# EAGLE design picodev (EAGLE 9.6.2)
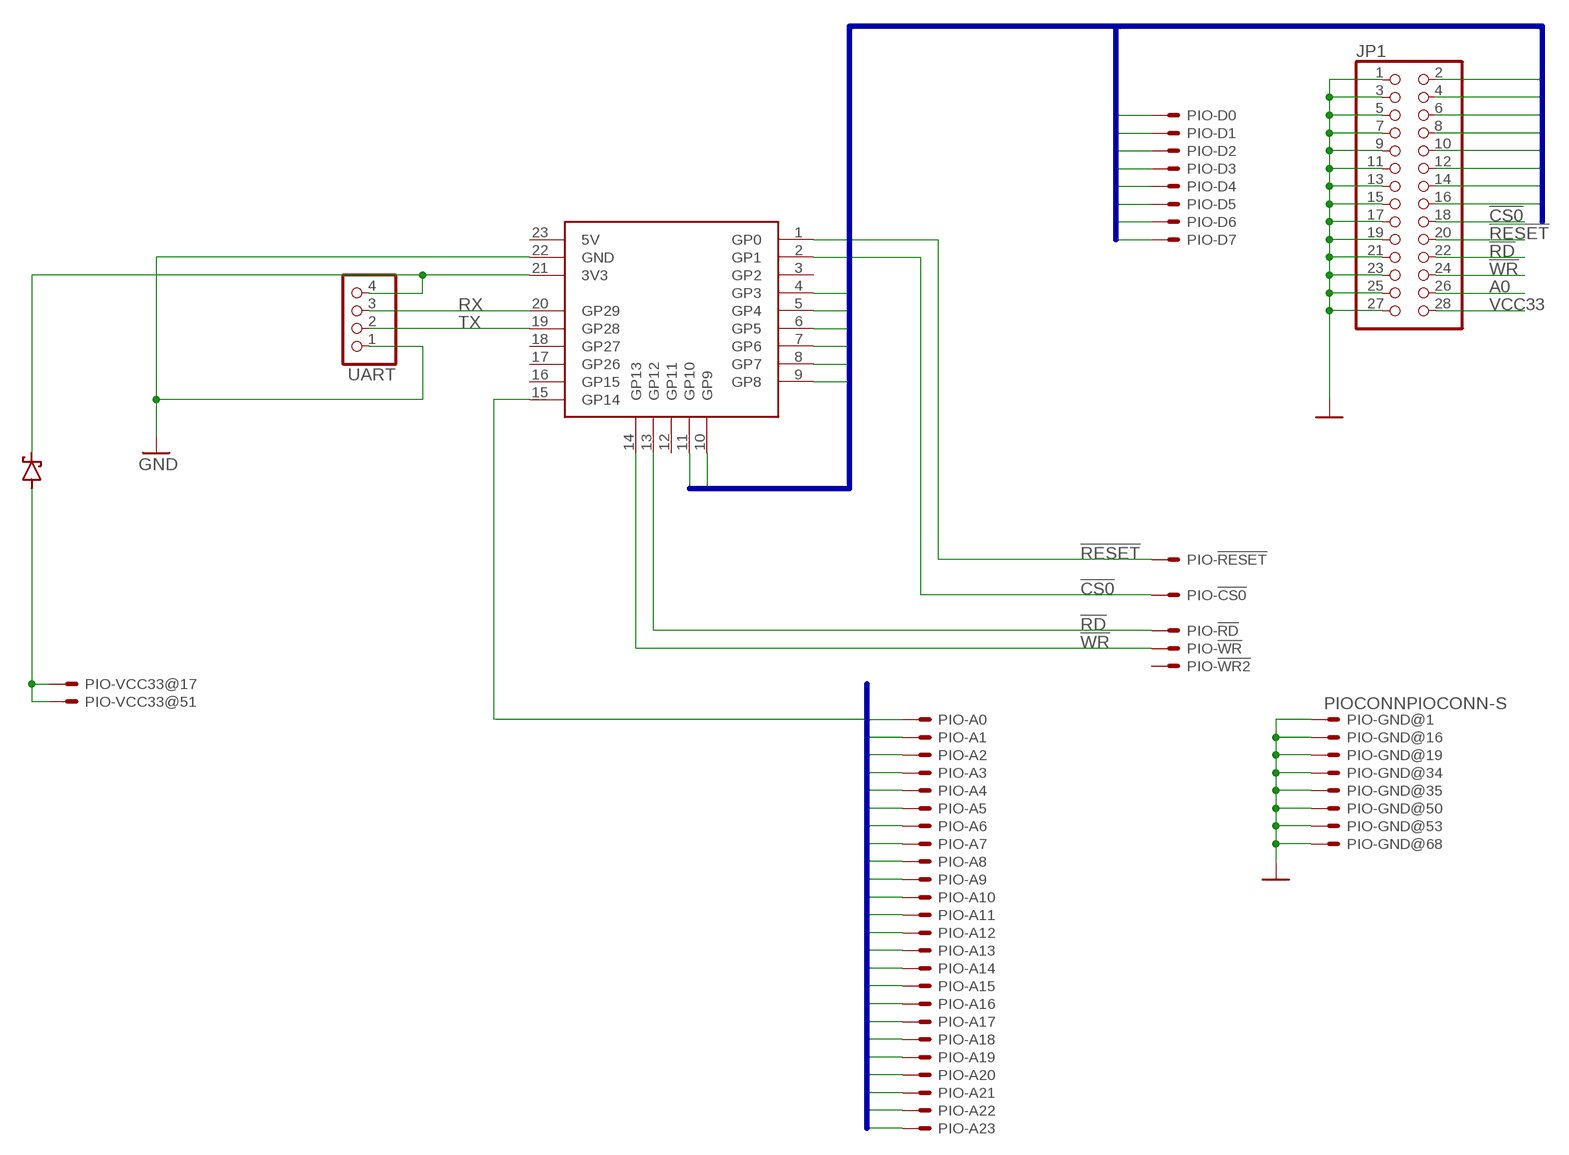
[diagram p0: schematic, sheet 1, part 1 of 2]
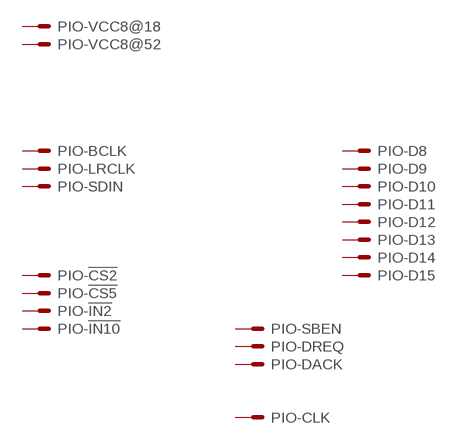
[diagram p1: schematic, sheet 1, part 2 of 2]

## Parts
D  SCHOTTKYSMA  [SMADIODE]
JP1  PINHD-2X14  [2X14]
PIO  PIOCONNPIOCONN-S  [PIOCONN]
U$1  PICO-ZERO  [PICO-ZERO]
UART  PINHD-1X4  [1X04]

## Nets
!CS0: JP1.18 PIO.4 U$1.2(GP1)
!RD: JP1.22 PIO.30 U$1.13(GP12)
!RESET: JP1.20 PIO.2 U$1.1(GP0)
!WR: JP1.24 PIO.64 U$1.14(GP13)
A0: JP1.26 PIO.14 U$1.15(GP14)
A1: PIO.48
A2: PIO.15
A3: PIO.49
A4: PIO.20
A5: PIO.54
A6: PIO.21
A7: PIO.55
A8: PIO.22
A9: PIO.56
A10: PIO.23
A11: PIO.57
A12: PIO.24
A13: PIO.58
A14: PIO.25
A15: PIO.59
A16: PIO.26
A17: PIO.60
A18: PIO.27
A19: PIO.61
A20: PIO.28
A21: PIO.62
A22: PIO.29
A23: PIO.63
D0: JP1.16 PIO.6 U$1.4(GP3)
D1: JP1.14 PIO.40 U$1.5(GP4)
D2: JP1.12 PIO.7 U$1.6(GP5)
D3: JP1.10 PIO.41 U$1.7(GP6)
D4: JP1.8 PIO.8 U$1.8(GP7)
D5: JP1.6 PIO.42 U$1.9(GP8)
D6: JP1.4 PIO.9 U$1.10(GP9)
D7: JP1.2 PIO.43 U$1.11(GP10)
GND: JP1.1 JP1.3 JP1.5 JP1.7 JP1.9 JP1.11 JP1.13 JP1.15 JP1.17 JP1.19 JP1.21 JP1.23 JP1.25 JP1.27 PIO.1 PIO.16 PIO.19 PIO.34 PIO.35 PIO.50 PIO.53 PIO.68 U$1.22(GND) UART.1
PIOVCC33: D.A PIO.17 PIO.51
RX: U$1.20(GP29) UART.3
TX: U$1.19(GP28) UART.2
VCC33: D.C JP1.28 U$1.21(3V3) UART.4
Unconnected: PIO.3 PIO.5 PIO.10 PIO.11 PIO.12 PIO.13 PIO.18 PIO.31 PIO.32 PIO.33 PIO.36 PIO.37 PIO.38 PIO.39 PIO.44 PIO.45 PIO.46 PIO.47 PIO.52 PIO.65 PIO.66 PIO.67 U$1.3(GP2) U$1.12(GP11) U$1.16(GP15) U$1.17(GP26) U$1.18(GP27) U$1.23(5V)

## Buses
A[0..23]
D[0..7]

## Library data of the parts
D = pixel:SCHOTTKY
JP1 = pinhead:PINHD-2X14: PIN HEADER
PIO = pixel:PIOCONN: CONNECTOR 68-pin 1.27mm (.050 inch) pitch SCSI+ unshielded receptacle right angle all plastic
U$1 = pixel:PICO-ZERO
UART = pinhead:PINHD-1X4: PIN HEADER

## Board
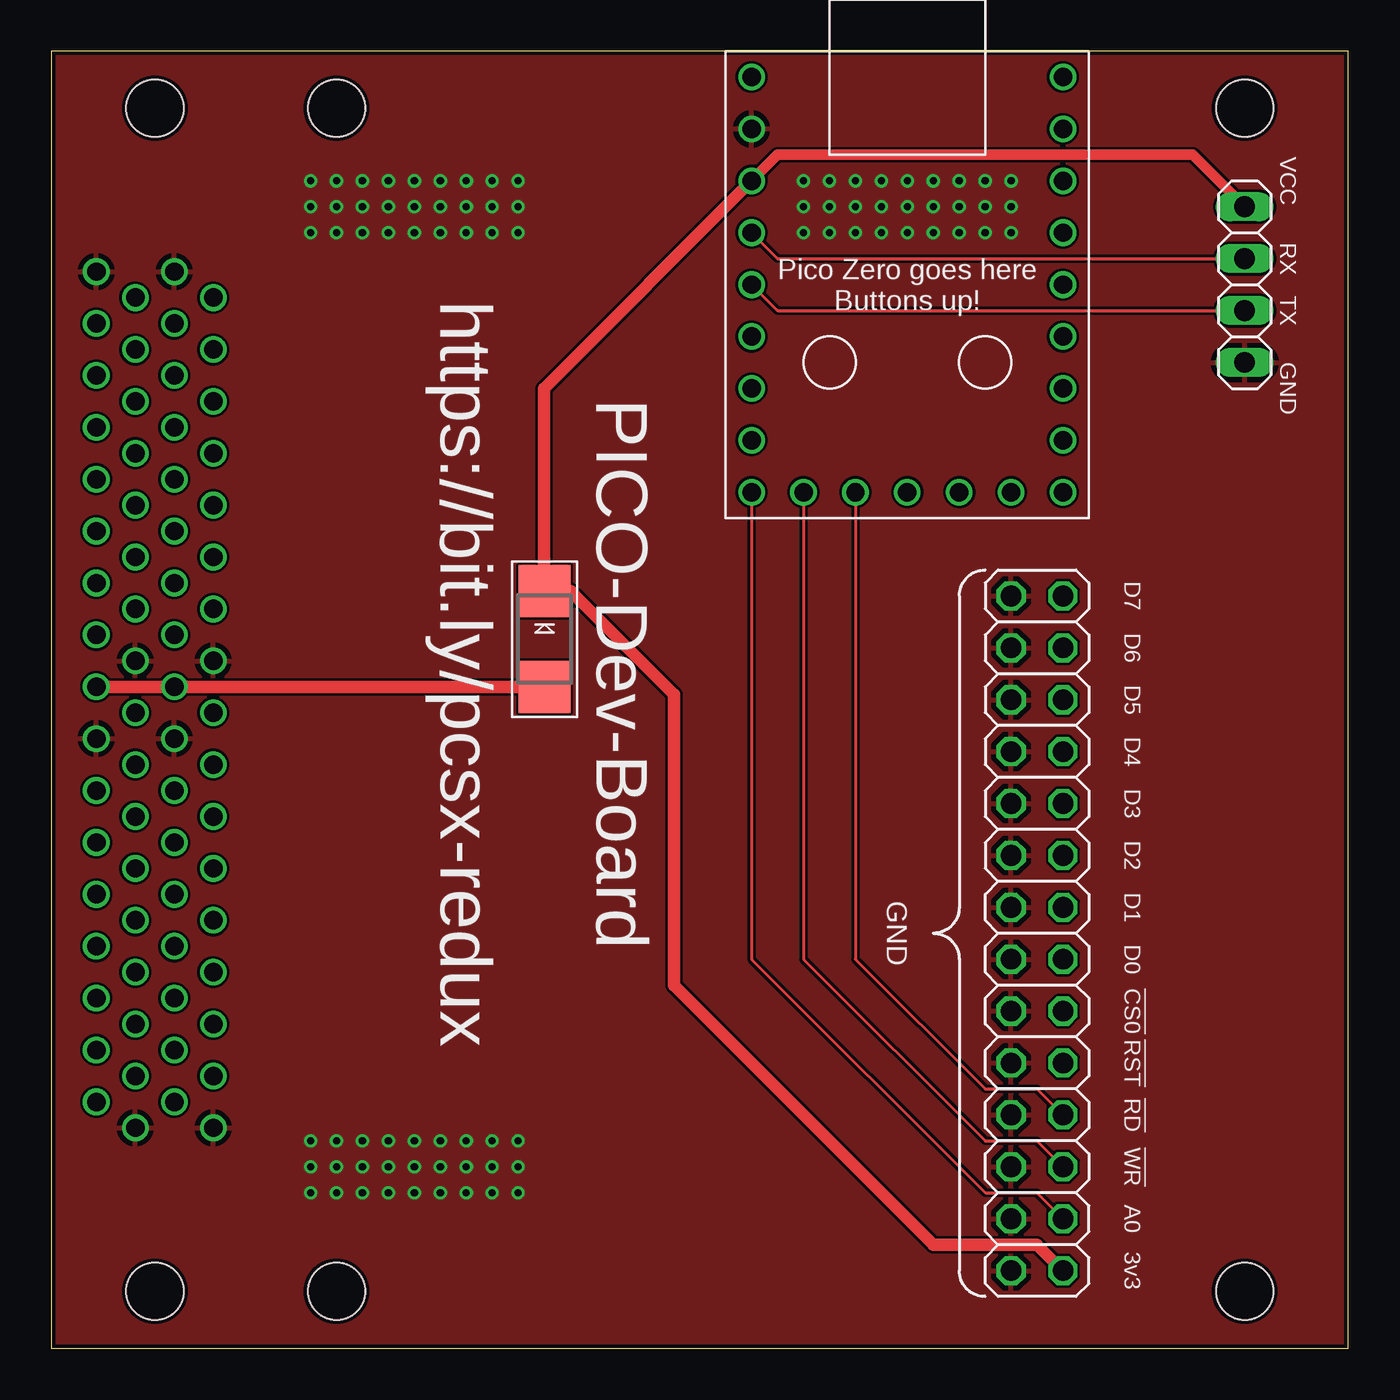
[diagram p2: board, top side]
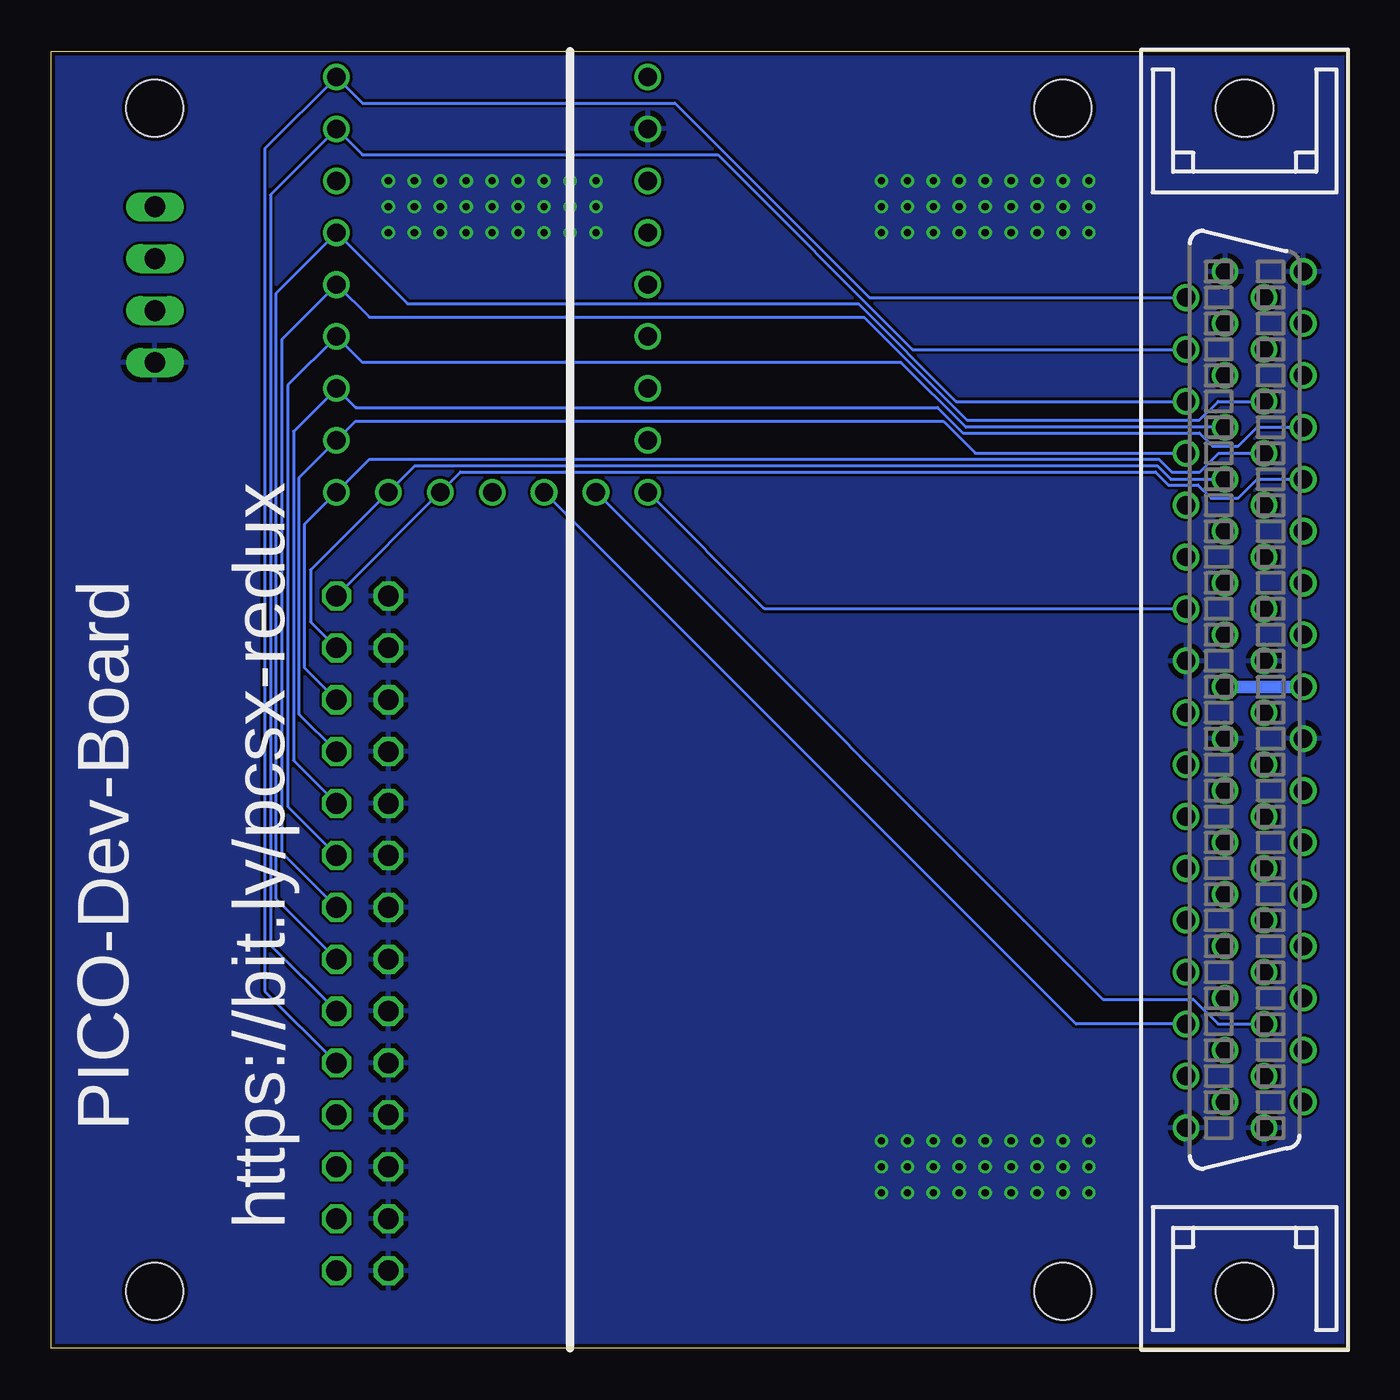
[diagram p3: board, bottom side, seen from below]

Size 63.5 x 63.5 mm. Coordinates in mm from the lower left corner, seen from the top.
Outline: 0,0 63.5,0 63.5,63.5 0,63.5 0,0
Copper layers (1*16): Top 0.035mm / dielectric 1.5mm / Bottom 0.035mm
Design rules "default *": minimum track width 5mil, minimum drill 0.2mm, track to track 5mil, track to pad 0.2mm, pad to pad 5mil, via to via 0.2mm, smd to smd 5mil, copper to edge 0.2mm, drill to drill 6mil, minimum pad ring 8mil, minimum via ring 0.15mm, stop-mask expansion 4mil, vias tented up to drill 25mil, thermal gap 10mil
Holes 2.79 mm at 58.42,60.71 58.42,2.79 13.97,60.71 13.97,2.79

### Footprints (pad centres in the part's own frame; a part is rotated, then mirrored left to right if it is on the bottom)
SMADIODE = smd 2.54 x 2.54: A 2.349,0; C -2.349,0
2X14 = drill 1.016 octagon: 1 -16.51,-1.27; 2 -16.51,1.27; 3 -13.97,-1.27; 4 -13.97,1.27; 5 -11.43,-1.27; 6 -11.43,1.27; 7 -8.89,-1.27; 8 -8.89,1.27; 9 -6.35,-1.27; 10 -6.35,1.27; 11 -3.81,-1.27; 12 -3.81,1.27; 13 -1.27,-1.27; 14 -1.27,1.27; 15 1.27,-1.27; 16 1.27,1.27; 17 3.81,-1.27; 18 3.81,1.27; 19 6.35,-1.27; 20 6.35,1.27; 21 8.89,-1.27; 22 8.89,1.27; 23 11.43,-1.27; 24 11.43,1.27; 25 13.97,-1.27; 26 13.97,1.27; 27 16.51,-1.27; 28 16.51,1.27
PIOCONN = drill 0.9 pad 1.27: 1 20.955,0.953; 2 19.685,2.863; 3 18.415,0.953; 4 17.145,2.863; 5 15.875,0.953; 6 14.605,2.863; 7 13.335,0.953; 8 12.065,2.863; 9 10.795,0.953; 10 9.525,2.863; 11 8.255,0.953; 12 6.985,2.863; 13 5.715,0.953; 14 4.445,2.863; 15 3.175,0.953; 16 1.905,2.863; 17 0.635,0.953; 18 -0.635,2.863; 19 -1.905,0.953; 20 -3.175,2.863; 21 -4.445,0.953; 22 -5.715,2.863; 23 -6.985,0.953; 24 -8.255,2.863; 25 -9.525,0.953; 26 -10.795,2.863; 27 -12.065,0.953; 28 -13.335,2.863; 29 -14.605,0.953; 30 -15.875,2.863; 31 -17.145,0.953; 32 -18.415,2.863; 33 -19.685,0.953; 34 -20.955,2.863; 35 20.955,-2.867; 36 19.685,-0.957; 37 18.415,-2.867; 38 17.145,-0.957; 39 15.875,-2.867; 40 14.605,-0.957; 41 13.335,-2.867; 42 12.065,-0.957; 43 10.795,-2.867; 44 9.525,-0.957; 45 8.255,-2.867; 46 6.985,-0.957; 47 5.715,-2.867; 48 4.445,-0.957; 49 3.175,-2.867; 50 1.905,-0.957; 51 0.635,-2.867; 52 -0.635,-0.957; 53 -1.905,-2.867; 54 -3.175,-0.957; 55 -4.445,-2.867; 56 -5.715,-0.957; 57 -6.985,-2.867; 58 -8.255,-0.957; 59 -9.525,-2.867; 60 -10.795,-0.957; 61 -12.065,-2.867; 62 -13.335,-0.957; 63 -14.605,-2.867; 64 -15.875,-0.957; 65 -17.145,-2.867; 66 -18.415,-0.957; 67 -19.685,-2.867; 68 -20.955,-0.957 | hole 2.8: -28.955,0; 28.955,0
PICO-ZERO = drill 0.9 pad 1.27: 1 7.62,10.16; 2 7.62,7.62; 3 7.62,5.08; 4 7.62,2.54; 5 7.62,0; 6 7.62,-2.54; 7 7.62,-5.08; 8 7.62,-7.62; 9 7.62,-10.16; 10 5.08,-10.16; 11 2.54,-10.16; 12 0,-10.16; 13 -2.54,-10.16; 14 -5.08,-10.16; 15 -7.62,-10.16; 16 -7.62,-7.62; 17 -7.62,-5.08; 18 -7.62,-2.54; 19 -7.62,0; 20 -7.62,2.54; 21 -7.62,5.08; 22 -7.62,7.62; 23 -7.62,10.16
1X04 = drill 1.016 long: 1 -3.81,0; 2 -1.27,0; 3 1.27,0; 4 3.81,0

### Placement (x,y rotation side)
D  24.16,34.72 270 top
JP1  48.26,20.32 270 top
PIO  5.08,31.75 90 bottom
U$1  41.91,52.07 0 top
UART  58.42,52.07 90 top

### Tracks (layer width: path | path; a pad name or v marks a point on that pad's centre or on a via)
!CS0
  Bottom 0.152: PIO.4 21.34,48.9 30.86,58.42 48.26,58.42 U$1.2 52.76,56.46 52.76,19.74 JP1.18
!RD
  Top 0.152: JP1.22 48.26,12.7 45.72,12.7 39.37,19.05 U$1.13
  Bottom 0.152: PIO.30 13.34,15.88 U$1.13
!RESET
  Bottom 0.152: PIO.2 23.44,51.44 32.97,60.96 48.26,60.96 U$1.1 53.03,58.73 53.03,17.48 JP1.20
!WR
  Top 0.152: U$1.14 36.83,19.05 45.72,10.16 48.26,10.16 JP1.24
  Bottom 0.152: U$1.14 12.01,17.09 7.59,17.09 6.38,15.88 PIO.64
A0
  Top 0.152: U$1.15 34.29,19.05 45.72,7.62 48.26,7.62 JP1.26
  Bottom 0.152: U$1.15 28.57,36.2 PIO.14
D0
  Bottom 0.152: PIO.6 19.2,46.35 23.98,51.13 46.05,51.13 U$1.4 52.48,51.66 52.48,22 JP1.16
D1
  Bottom 0.152: U$1.5 49.52,52.07 | 49.52,52.07 47.92,50.47 23.71,50.47 18.67,45.43 7.3,45.43 6.38,46.35 PIO.40 | JP1.14 52.2,24.26 52.2,49.39 49.52,52.07
D2
  Bottom 0.152: PIO.7 18.72,45.09 21.9,48.26 48.26,48.26 U$1.6 51.92,47.14 51.92,26.52 JP1.12
D3
  Bottom 0.152: PIO.41 4.46,45.09 5.39,44.16 6.64,44.16 7.29,44.81 18.86,44.81 20.11,46.05 48.59,46.05 U$1.7 51.64,44.88 51.64,28.78 JP1.10
D4
  Bottom 0.152: PIO.8 18.27,43.81 19.83,45.38 48.59,45.38 U$1.8 51.36,42.62 51.36,31.04 JP1.8
D5
  Bottom 0.152: PIO.42 6.35,43.81 7.28,42.89 8.63,42.89 9.27,43.52 47.92,43.52 U$1.9 51.08,40.36 51.08,33.3 JP1.6
D6
  Bottom 0.152: PIO.9 8.69,42.55 9.35,43.2 45.7,43.2 U$1.10 50.8,38.1 50.8,35.56 JP1.4
D7
  Bottom 0.152: PIO.43 4.47,42.55 5.4,41.62 6.72,41.62 7.37,42.27 8.81,42.27 9.44,42.9 43.46,42.9 U$1.11 JP1.2
GND  (via drill 0.35)
  other vias: 36.83,57.15 38.1,57.15 39.37,57.15 40.64,57.15 41.91,57.15 43.18,57.15 44.45,57.15 45.72,57.15 46.99,57.15 36.83,55.88 38.1,55.88 39.37,55.88 40.64,55.88 41.91,55.88 43.18,55.88 44.45,55.88 45.72,55.88 46.99,55.88 46.99,54.61 45.72,54.61 44.45,54.61 43.18,54.61 41.91,54.61 40.64,54.61 39.37,54.61 38.1,54.61 36.83,54.61 12.7,10.16 13.97,10.16 15.24,10.16 16.51,10.16 17.78,10.16 19.05,10.16 20.32,10.16 21.59,10.16 22.86,10.16 12.7,8.89 13.97,8.89 15.24,8.89 16.51,8.89 17.78,8.89 19.05,8.89 20.32,8.89 21.59,8.89 22.86,8.89 22.86,7.62 21.59,7.62 20.32,7.62 19.05,7.62 17.78,7.62 16.51,7.62 15.24,7.62 13.97,7.62 12.7,7.62 12.7,57.15 13.97,57.15 15.24,57.15 16.51,57.15 17.78,57.15 19.05,57.15 20.32,57.15 21.59,57.15 22.86,57.15 12.7,55.88 13.97,55.88 15.24,55.88 16.51,55.88 17.78,55.88 19.05,55.88 20.32,55.88 21.59,55.88 22.86,55.88 22.86,54.61 21.59,54.61 20.32,54.61 19.05,54.61 17.78,54.61 16.51,54.61 15.24,54.61 13.97,54.61 12.7,54.61
  pour Top: 0,63.5 63.5,63.5 63.5,0 0,0
  pour Bottom: 0,63.5 63.5,63.5 63.5,0 0,0
PIOVCC33
  Top 0.61: PIO.51 PIO.17 24.14,32.38 D.A
  Bottom 0.61: PIO.51 5.97,32.38
RX
  Top 0.152: U$1.20 35.56,53.34 UART.3
TX
  Top 0.152: U$1.19 35.56,50.8 UART.2
VCC33
  Top 0.508: U$1.21 35.55,58.42 55.88,58.42 UART.4
  Top 0.61: U$1.21 24.13,46.99 24.13,37.1 D.C 25.43,37.07 30.48,32.02 30.48,17.78 43.18,5.08 48.26,5.08 JP1.28

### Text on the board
tPlace: Pico Zero goes here / Buttons up! | GND
tNames: VCC | RX | TX | GND | D7 | D6 | PICO-Dev-Board / / https://bit.ly/pcsx-redux | D5 | D4 | D3 | D2 | D1 | D0 | !CS0 | !RST | !RD | !WR | A0 | 3v3
bNames: PICO-Dev-Board / / https://bit.ly/pcsx-redux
